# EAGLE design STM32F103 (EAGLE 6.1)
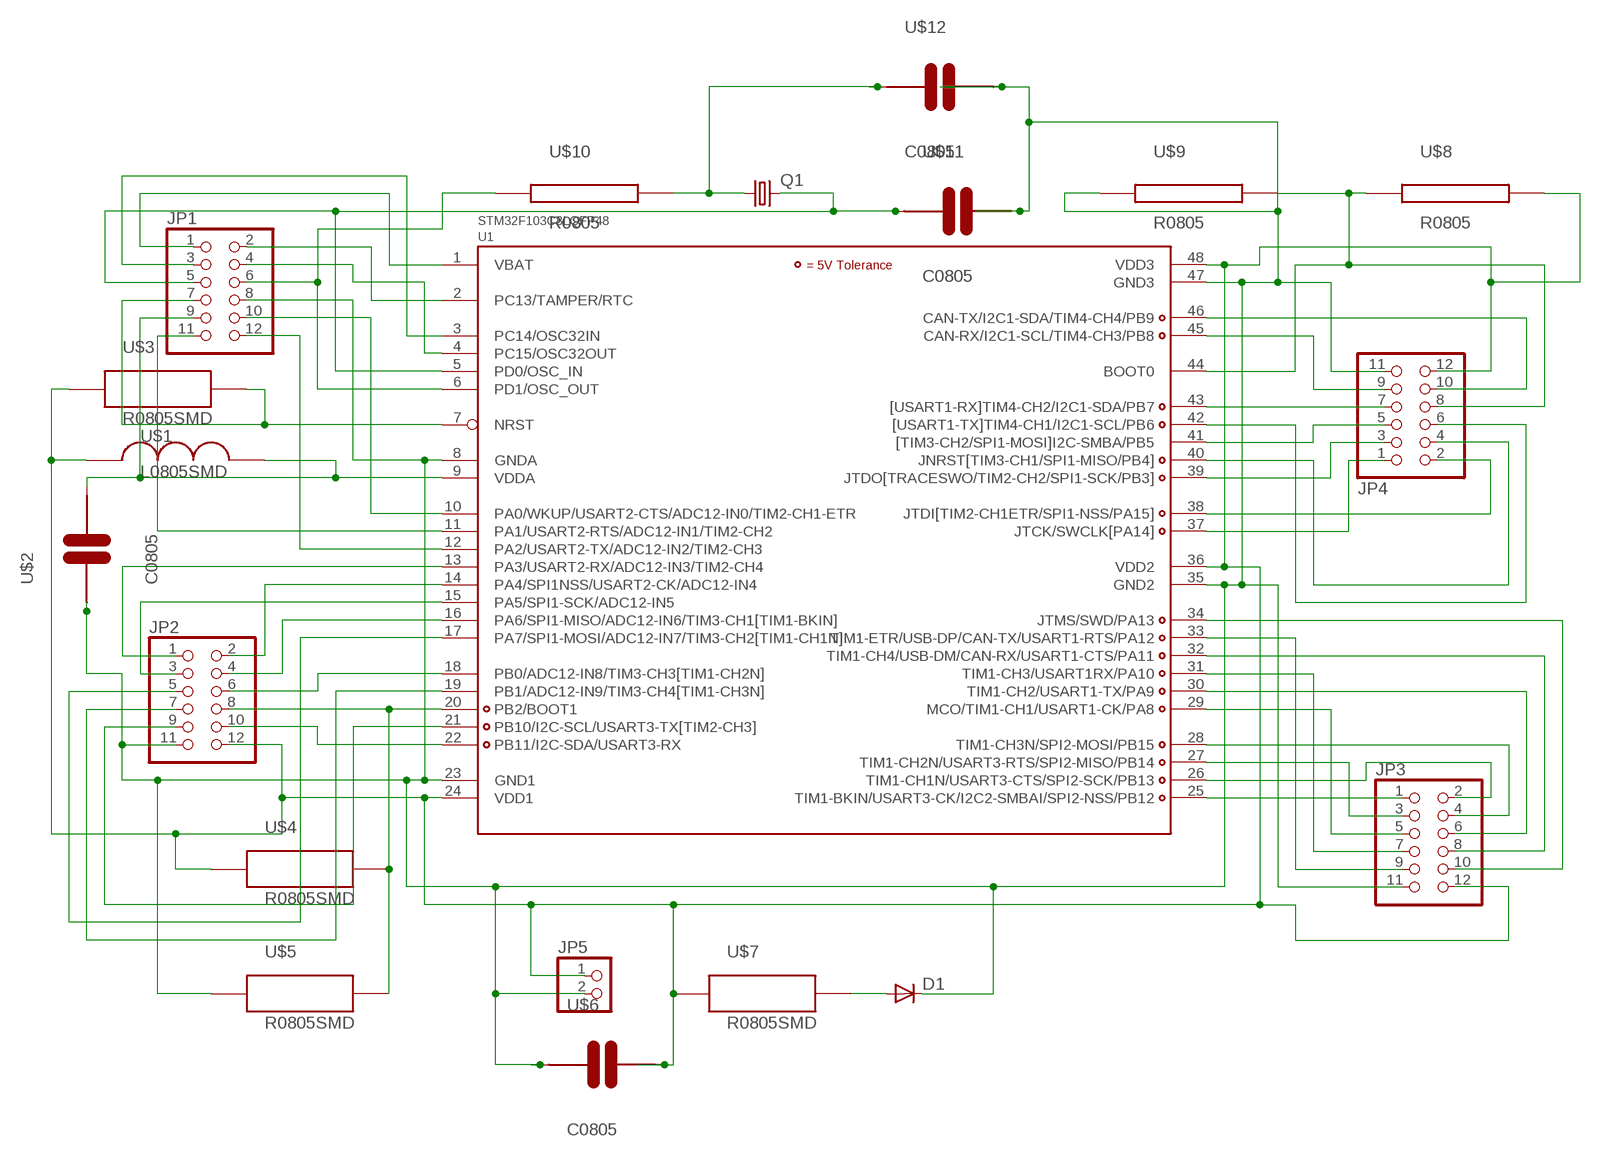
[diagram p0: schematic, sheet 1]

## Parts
D1  DIODE-DO214BA  [DO214BA]
JP1  PINHD-2X6  [2X06]
JP2  PINHD-2X6  [2X06]
JP3  PINHD-2X6  [2X06]
JP4  PINHD-2X6  [2X06]
JP5  PINHD-1X2  [1X02]
Q1  CRYSTALHC49U70  [HC49U70]
U1  STM32F103C8LQFP48  [LQFP48]
U$1  L0805SMD  [SMD0805]
U$2  C0805  [C0805]
U$3  R0805SMD  [SMD0805]
U$4  R0805SMD  [SMD0805]
U$5  R0805SMD  [SMD0805]
U$6  C0805  [C0805]
U$7  R0805SMD  [SMD0805]
U$8  R0805  [SMD0805]
U$9  R0805  [SMD0805]
U$10  R0805  [SMD0805]
U$11  C0805  [C0805]
U$12  C0805  [C0805]

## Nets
N$1: JP2.1 U1.13(PA3/USART2-RX/ADC12-IN3/TIM2-CH4)
N$2: JP1.2 U1.2(PC13/TAMPER/RTC)
N$3: JP1.3 U1.3(PC14/OSC32IN)
N$4: JP1.4 U1.4(PC15/OSC32OUT)
N$5: JP1.5 Q1.2 U1.5(PD0/OSC_IN) U$11.1
N$6: JP1.6 U1.6(PD1/OSC_OUT) U$10.1
N$7: JP1.7 U1.7(NRST) U$3.2
N$8: JP1.10 U1.10(PA0/WKUP/USART2-CTS/ADC12-IN0/TIM2-CH1-ETR)
N$9: JP1.11 U1.11(PA1/USART2-RTS/ADC12-IN1/TIM2-CH2)
N$10: JP1.12 U1.12(PA2/USART2-TX/ADC12-IN2/TIM2-CH3)
N$11: JP2.2 U1.14(PA4/SPI1NSS/USART2-CK/ADC12-IN4)
N$12: JP2.3 U1.15(PA5/SPI1-SCK/ADC12-IN5)
N$13: JP2.4 U1.16(PA6/SPI1-MISO/ADC12-IN6/TIM3-CH1[TIM1-BKIN])
N$14: JP2.5 U1.17(PA7/SPI1-MOSI/ADC12-IN7/TIM3-CH2[TIM1-CH1N])
N$15: JP2.6 U1.18(PB0/ADC12-IN8/TIM3-CH3[TIM1-CH2N])
N$16: JP2.7 U1.19(PB1/ADC12-IN9/TIM3-CH4[TIM1-CH3N])
N$17: JP2.8 U1.20(PB2/BOOT1) U$4.2 U$5.2
N$18: JP2.9 U1.21(PB10/I2C-SCL/USART3-TX[TIM2-CH3])
N$19: JP2.10 U1.22(PB11/I2C-SDA/USART3-RX)
N$20: JP3.1 U1.25(TIM1-BKIN/USART3-CK/I2C2-SMBAI/SPI2-NSS/PB12)
N$21: JP3.2 U1.26(TIM1-CH1N/USART3-CTS/SPI2-SCK/PB13)
N$22: JP3.3 U1.27(TIM1-CH2N/USART3-RTS/SPI2-MISO/PB14)
N$23: JP3.4 U1.28(TIM1-CH3N/SPI2-MOSI/PB15)
N$24: JP3.5 U1.29(MCO/TIM1-CH1/USART1-CK/PA8)
N$25: JP3.6 U1.30(TIM1-CH2/USART1-TX/PA9)
N$26: JP3.7 U1.31(TIM1-CH3/USART1RX/PA10)
N$27: JP3.8 U1.32(TIM1-CH4/USB-DM/CAN-RX/USART1-CTS/PA11)
N$28: JP3.9 U1.33(TIM1-ETR/USB-DP/CAN-TX/USART1-RTS/PA12)
N$29: JP3.10 U1.34(JTMS/SWD/PA13)
N$30: JP4.1 U1.37(JTCK/SWCLK[PA14])
N$31: JP4.2 U1.38(JTDI[TIM2-CH1ETR/SPI1-NSS/PA15])
N$32: JP4.3 U1.39(JTDO[TRACESWO/TIM2-CH2/SPI1-SCK/PB3])
N$33: JP4.4 U1.40(JNRST[TIM3-CH1/SPI1-MISO/PB4])
N$34: JP4.5 U1.41([TIM3-CH2/SPI1-MOSI]I2C-SMBA/PB5)
N$35: JP4.6 U1.42([USART1-TX]TIM4-CH1/I2C1-SCL/PB6)
N$36: JP4.7 U1.43([USART1-RX]TIM4-CH2/I2C1-SDA/PB7)
N$37: JP4.8 U1.44(BOOT0) U$8.1 U$9.2
N$38: JP4.9 U1.45(CAN-RX/I2C1-SCL/TIM4-CH3/PB8)
N$39: JP4.10 U1.46(CAN-TX/I2C1-SDA/TIM4-CH4/PB9)
N$50: Q1.1 U$10.2 U$12.1
N$54: D1.A U$7.2
N$68: JP2.12 JP3.12 JP4.12 JP5.1 U1.24(VDD1) U1.36(VDD2) U1.48(VDD3) U$1.1 U$3.1 U$4.1 U$6.2 U$7.1 U$8.2
N$80: D1.C JP1.8 JP2.11 JP3.11 JP4.11 JP5.2 U1.8(GNDA) U1.23(GND1) U1.35(GND2) U1.47(GND3) U$2.1 U$5.1 U$6.1 U$9.1 U$11.2 U$12.2
VBAT: JP1.1 U1.1(VBAT)
VDDA: JP1.9 U1.9(VDDA) U$1.2 U$2.2

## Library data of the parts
D1 = diode:DIODE-: DIODE
JP1-JP4 = pinhead:PINHD-2X6: PIN HEADER
JP5 = pinhead:PINHD-1X2: PIN HEADER
Q1 = crystal:CRYSTAL: CRYSTAL
U1 = STM32:STM32F103C8
U$1 = cansat1:L0805SMD: indukcnost v provedeni SMD0805
U$2 U$6 U$11 U$12 = cansat1:C0805: kondenzator v provedeni SMD0805
U$3-U$5 U$7 = cansat1:R0805SMD: REZISTOR v provedeni SMD0805
U$8-U$10 = cansat1:R0805: REZISTOR v provedeni SMD0805

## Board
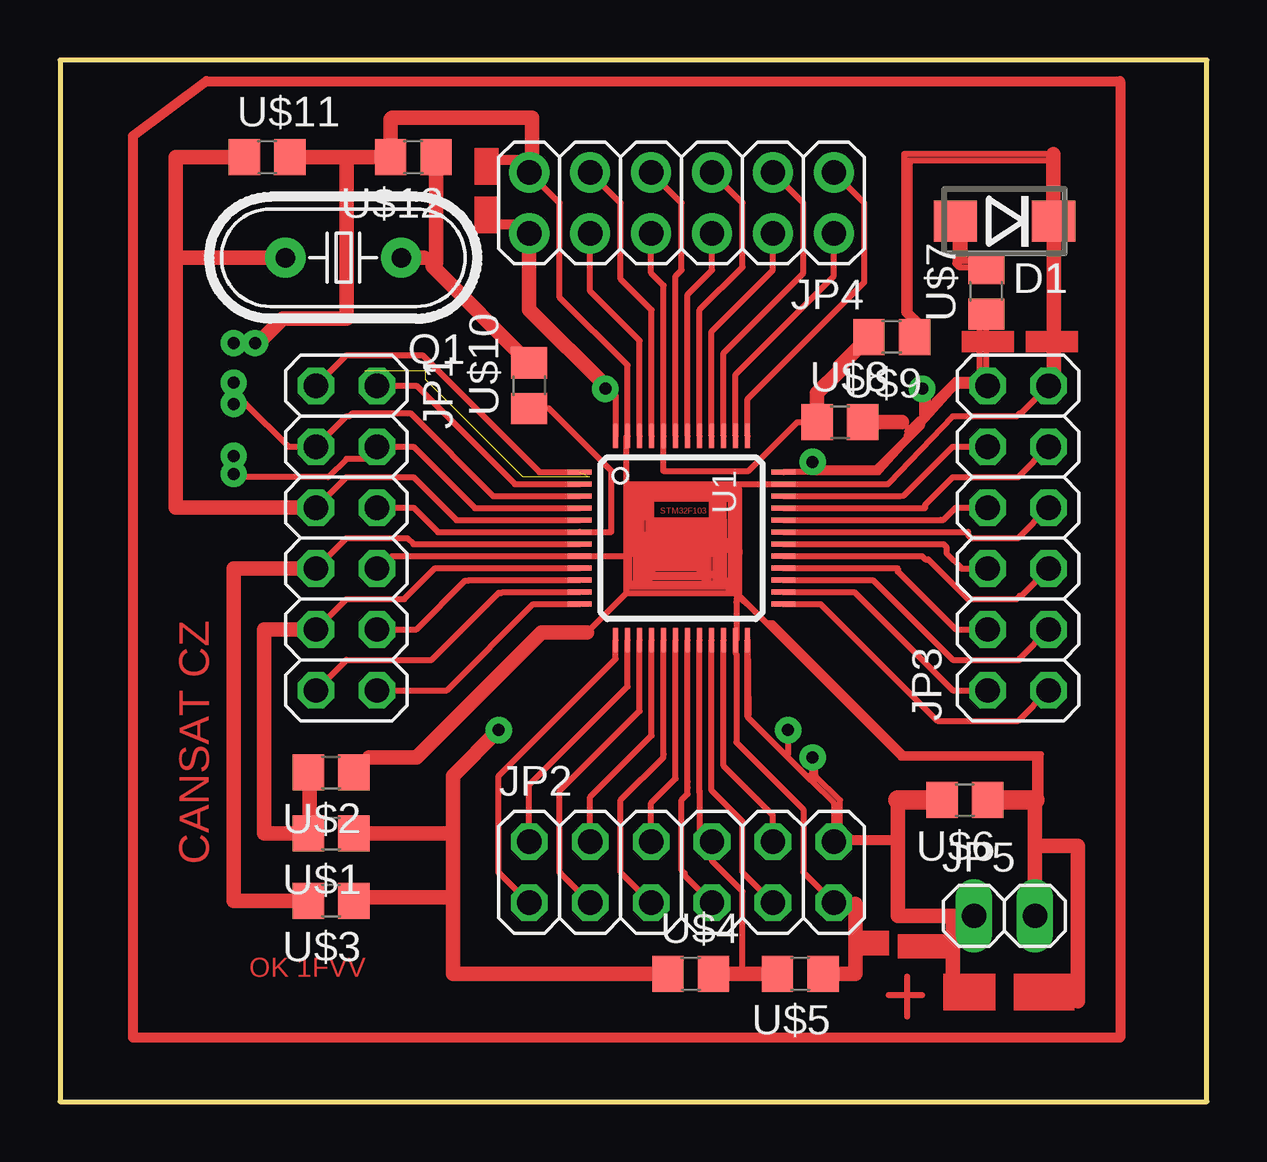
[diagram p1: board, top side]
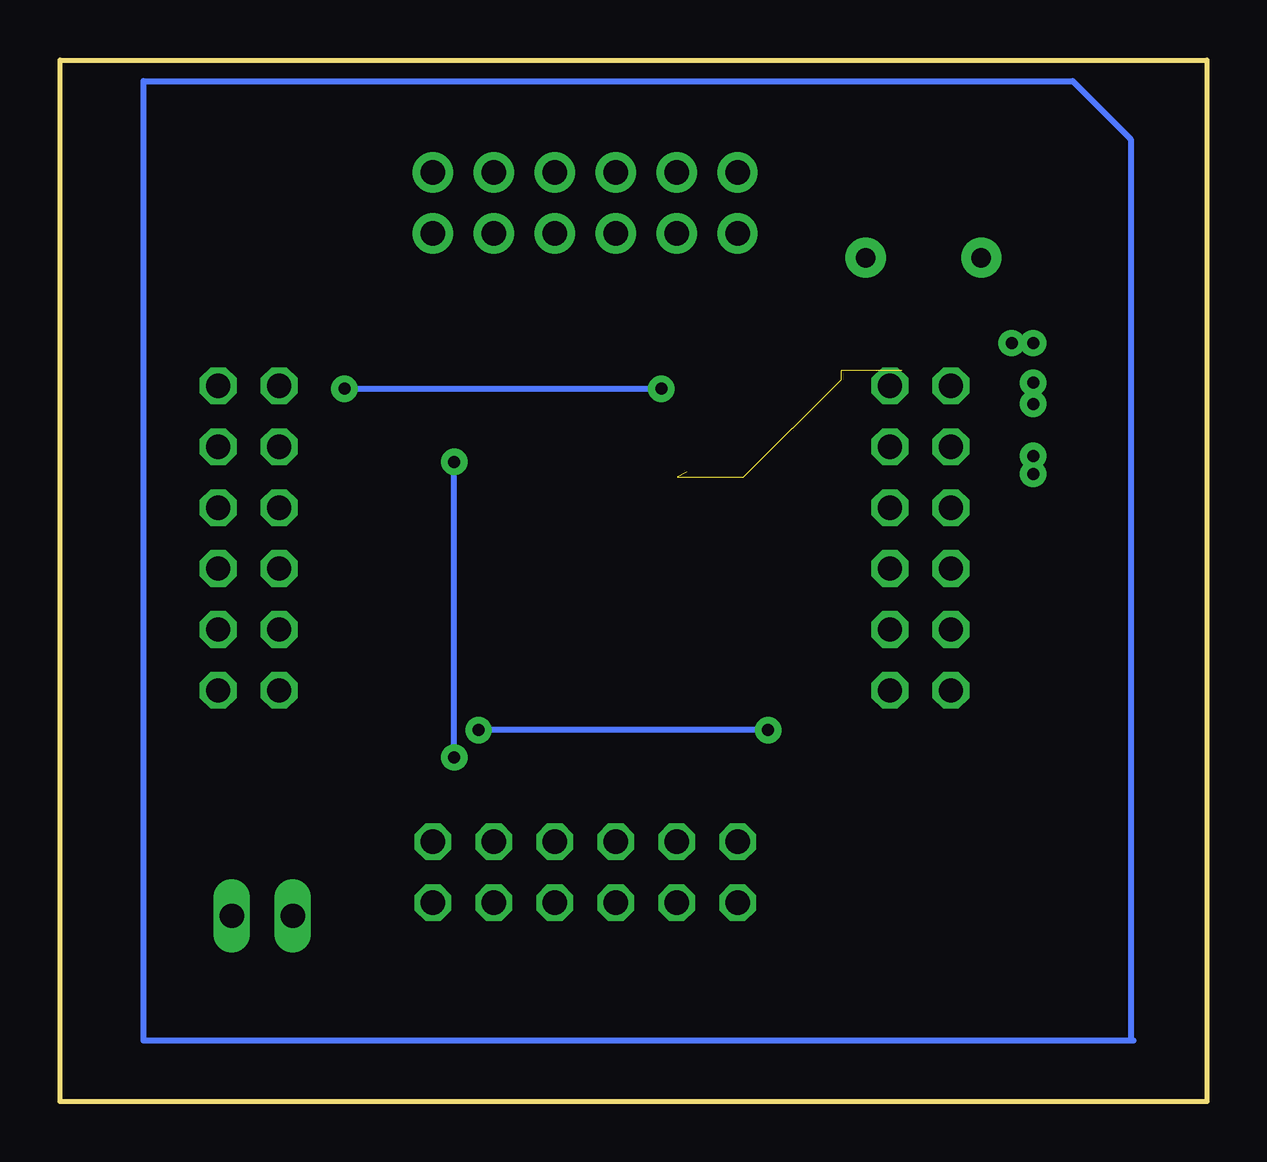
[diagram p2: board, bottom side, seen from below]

Size 47.8 x 43.42 mm. Coordinates in mm from the lower left corner, seen from the top.
Outline: 0,0 47.8,0 47.8,43.42 0,43.42 0,0
Copper layers (1*16): Top 0.035mm / dielectric 1.5mm / Bottom 0.035mm
Design rules: minimum track width 0.2mm, minimum drill 0.6mm, track to track 0.2mm, track to pad 0.2mm, pad to pad 0.2mm, via to via 0.2mm, smd to smd 8mil, copper to edge 40mil, drill to drill 2mm, minimum pad ring 0.2mm, minimum via ring 0.3mm, stop-mask expansion 4mil, vias tented up to drill 0mil, thermal gap 10mil

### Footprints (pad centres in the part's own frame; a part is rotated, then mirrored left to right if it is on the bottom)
DO214BA = smd 1.8 x 1.7: A 2.05,0; C -2.05,0
2X06 = drill 1.016 octagon: 1 -6.35,-1.27; 2 -6.35,1.27; 3 -3.81,-1.27; 4 -3.81,1.27; 5 -1.27,-1.27; 6 -1.27,1.27; 7 1.27,-1.27; 8 1.27,1.27; 9 3.81,-1.27; 10 3.81,1.27; 11 6.35,-1.27; 12 6.35,1.27
1X02 = drill 1.016 long: 1 -1.27,0; 2 1.27,0
HC49U70 = drill 0.813: 1 -2.413,0; 2 2.413,0
LQFP48 = smd 0.2 x 1: 1 -2.75,-4.25; 2 -2.25,-4.25; 3 -1.75,-4.25; 4 -1.25,-4.25; 5 -0.75,-4.25; 6 -0.25,-4.25; 7 0.25,-4.25; 8 0.75,-4.25; 9 1.25,-4.25; 10 1.75,-4.25; 11 2.25,-4.25; 12 2.75,-4.25; 25 2.75,4.25; 26 2.25,4.25; 27 1.75,4.25; 28 1.25,4.25; 29 0.75,4.25; 30 0.25,4.25; 31 -0.25,4.25; 32 -0.75,4.25; 33 -1.25,4.25; 34 -1.75,4.25; 35 -2.25,4.25; 36 -2.75,4.25 | smd 1 x 0.2: 13 4.25,-2.75; 14 4.25,-2.25; 15 4.25,-1.75; 16 4.25,-1.25; 17 4.25,-0.75; 18 4.25,-0.25; 19 4.25,0.25; 20 4.25,0.75; 21 4.25,1.25; 22 4.25,1.75; 23 4.25,2.25; 24 4.25,2.75; 37 -4.25,2.75; 38 -4.25,2.25; 39 -4.25,1.75; 40 -4.25,1.25; 41 -4.25,0.75; 42 -4.25,0.25; 43 -4.25,-0.25; 44 -4.25,-0.75; 45 -4.25,-1.25; 46 -4.25,-1.75; 47 -4.25,-2.25; 48 -4.25,-2.75
SMD0805 = smd 1.3 x 1.5: 1 -0.95,0; 2 0.95,0
C0805 = smd 1.3 x 1.5: 1 -0.95,0; 2 0.95,0

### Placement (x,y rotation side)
D1  39.37,36.7 180 top
JP1  11.94,23.49 270 top
JP2  25.91,9.56 0 top
JP3  39.94,23.49 90 top
JP4  25.91,37.46 180 top
JP5  39.37,7.75 0 top
Q1  11.81,35.18 180 top
U1  25.91,23.49 270 top
U$1  11.3,11.18 180 top
U$2  11.3,13.72 180 top
U$3  11.3,8.38 180 top
U$4  26.29,5.33 0 top
U$5  30.86,5.33 180 top
U$6  37.72,12.57 180 top
U$7  38.61,33.78 90 top
U$8  32.51,28.32 0 top
U$9  34.67,31.88 180 top
U$10  19.56,29.84 90 top
U$11  8.64,39.37 0 top
U$12  14.73,39.37 180 top

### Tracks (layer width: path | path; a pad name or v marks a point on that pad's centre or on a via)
N$1
  Top 0.254: JP2.1 18.33,9.53 18.29,9.53 18.29,13.59 23.16,18.46 U1.13
N$2
  Top 0.254: JP1.2 14.86,29.84 18.96,25.74 U1.2
N$3
  Top 0.254: JP1.3 11.94,28.57 12.06,28.57 12.19,28.7 14.61,28.7 18.06,25.24 U1.3
N$4
  Top 0.254: U1.4 17.29,24.74 14.73,27.3 JP1.4 12.7,26.8 11.94,26.8 11.18,26.03 7.62,26.03
N$5
  Top 0.254: JP1.5 11.94,26.03 14.73,26.03 16.52,24.24 U1.5
  Top 0.61: 4.83,35.18 Q1.2 | 4.83,35.18 4.83,24.77 JP1.5 | 4.83,35.18 4.83,39.37 U$11.1
N$6
  Top 0.254: JP1.6 14.73,24.77 15.75,23.74 U1.6 22.99,23.75 22.99,26.29 20.38,28.89 U$10.1
N$7
  Top 0.254: JP1.7 11.94,23.49 14.48,23.49 14.73,23.24 15.37,23.24 U1.7
  Top 0.61: JP1.7 7.24,22.23 7.24,8.38 U$3.2
N$8
  Top 0.254: JP1.10 14.86,19.69 16.89,21.72 17.02,21.72 17.05,21.74 U1.10
N$9
  Top 0.254: JP1.11 11.94,18.41 15.49,18.41 18.29,21.21 18.41,21.21 18.45,21.24 U1.11
N$10
  Top 0.254: JP1.12 16.13,17.14 19.73,20.74 U1.12
N$11
  Top 0.254: JP2.2 19.56,13.21 23.66,17.31 U1.14
N$12
  Top 0.254: JP2.3 20.87,9.53 20.83,9.53 20.83,12.95 24.16,16.28 U1.15
N$13
  Top 0.254: JP2.4 22.1,12.7 24.66,15.26 U1.16
N$14
  Top 0.254: JP2.5 23.37,9.56 23.37,12.57 25.15,14.35 25.15,14.48 25.16,14.49 U1.17
N$15
  Top 0.254: JP2.6 24.64,12.45 25.66,13.47 U1.18
N$16
  Top 0.254: U1.19 26.16,13.33 26.16,13.08 26.16,12.83 25.91,12.57 25.91,9.65 26.04,9.53 26.04,9.44 JP2.7
N$17
  Top 0.254: 26.67,11.47 JP2.8 | 26.67,11.47 26.67,12.83 26.66,12.94 U1.20 | 26.67,11.47 26.67,11.3 27.18,10.79 27.18,10.03 28.45,8.76 28.45,5.33
  Top 0.61: U$4.2 28.45,5.33 U$5.2
N$18
  Top 0.254: JP2.9 28.45,9.56 28.45,11.68 27.16,12.97 U1.21
N$19
  Top 0.254: JP2.10 29.72,11.94 27.66,14 U1.22
N$20
  Top 0.254: JP3.1 39.94,15.87 36.58,15.87 31.71,20.74 U1.25
N$21
  Top 0.254: JP3.2 37.21,17.14 33.11,21.24 U1.26
N$22
  Top 0.254: JP3.3 40.01,18.48 40.01,18.41 37.21,18.41 33.88,21.74 U1.27
N$23
  Top 0.254: JP3.4 37.34,19.69 34.92,22.1 34.92,22.23 34.91,22.24 U1.28
N$24
  Top 0.254: JP3.5 40.06,21.08 40.01,21.08 39.88,20.95 37.85,20.95 36.2,22.61 36.07,22.61 35.93,22.74 U1.29
N$25
  Top 0.254: JP3.6 37.59,22.23 36.96,22.86 36.96,23.11 36.83,23.24 U1.30
N$26
  Top 0.254: JP3.7 39.94,23.49 37.97,23.49 37.85,23.62 37.85,23.75 37.84,23.74 U1.31
N$27
  Top 0.254: JP3.8 37.34,24.77 36.83,24.26 36.7,24.26 36.69,24.24 U1.32
N$28
  Top 0.254: JP3.9 39.94,26.03 37.21,26.03 36.07,24.89 36.07,24.77 36.05,24.74 U1.33
N$29
  Top 0.254: JP3.10 37.21,27.3 35.18,25.27 35.02,25.24 U1.34
N$30
  Top 0.254: JP4.1 33.53,37.46 33.53,34.16 28.66,29.29 U1.37
N$31
  Top 0.254: JP4.2 32.26,34.42 28.16,30.32 U1.38
N$32
  Top 0.254: JP4.3 30.99,37.46 30.99,34.54 27.66,31.21 U1.39
N$33
  Top 0.254: JP4.4 29.72,34.67 27.16,32.11 U1.40
N$34
  Top 0.254: JP4.5 28.45,37.46 28.45,34.8 26.66,33.01 U1.41
N$35
  Top 0.254: JP4.6 27.18,34.67 26.16,33.65 U1.42
N$36
  Top 0.254: JP4.7 25.91,37.46 25.91,34.67 25.66,34.42 U1.43
N$37
  Top 0.254: JP4.8 24.64,34.54 25.16,34.02 U1.44 25.16,26.3 25.15,26.29 28.7,26.29 30.73,28.32 U$8.1 | 32.51,30.48 32.51,30.67
  Top 0.61: U$8.1 31.56,29.53 32.51,30.48 | 32.51,30.67 U$9.2
N$38
  Top 0.254: JP4.9 23.37,37.46 23.37,34.29 24.66,33 U1.45
N$39
  Top 0.254: JP4.10 22.1,33.78 24.16,31.72 U1.46
N$40  (via drill 0.7 pad 1.68)
  other vias: 19.56,36.2
N$41
  Top 0.254: 24.13,23.62 27.56,23.62 27.56,23.49 24.51,23.49 | 24.51,23.49 24.13,23.49 | 24.51,24.26 24.51,23.49 | 24.51,24.26 24.51,25.02 24.64,25.02 24.64,23.75 | 23.88,25.53 23.88,25.65 23.75,25.65 23.75,23.11 23.88,23.11 23.88,25.4 | 23.88,25.53 28.19,25.53 28.19,23.11 28.07,23.11 28.07,25.27 24,25.27 | 23.88,25.4 23.88,25.53 | 24,25.4 24.26,25.4 | 24,25.4 23.88,25.4 | 24,25.27 24,25.4 | 24,25.27 24,23.11 27.94,23.11 27.94,25.15 24.26,25.15 24.26,23.24 27.81,23.24 27.81,23.37 27.69,23.37 27.69,24.26 | 27.69,24.26 27.69,25.02 | 24.51,24.26 27.18,24.26 | 27.18,24.26 27.69,24.26 | 27.18,24.26 27.18,25.02 27.3,25.02 | 27.3,25.02 27.56,25.02 | 27.3,25.02 27.3,24.38 27.56,24.38 | 27.56,24.38 27.56,24.89 | 27.56,24.38 27.56,23.75 24.89,23.75 24.89,24.13 27.43,24.13 27.43,23.88 25.02,23.88 25.02,24 25.15,24
N$42
  Top 0.254: 24.51,23.37 27.43,23.37
N$43  (via drill 0.7 pad 1.68)
  other vias: 29.72,36.2
N$44  (via drill 0.7 pad 1.68)
  other vias: 24.64,36.2
N$45  (via drill 0.7 pad 1.68)
  other vias: 32.26,36.2
N$46  (via drill 0.7 pad 1.68)
  other vias: 27.18,36.2
N$47  (via drill 0.7 pad 1.68)
  other vias: 22.1,36.2
N$48  (via drill 0.7 pad 1.68)
  other vias: 9.4,35.18
N$49  (via drill 0.7 pad 1.68)
  other vias: 19.56,38.73
N$50
  Top 0.254: 15.17,35.18 15.52,34.83 15.68,34.99
  Top 0.61: Q1.1 15.17,35.18 | 15.52,34.83 U$10.2 | 15.68,34.99 U$12.1
N$51  (via drill 0.7 pad 1.68)
  other vias: 22.1,38.73
N$52  (via drill 0.7 pad 1.68)
  other vias: 24.64,38.73
N$53  (via drill 0.5 pad 0.81)
  other vias: 7.24,26.16
N$54
  Top 0.254: D1.A 37.32,34.94 37.46,34.8 38.54,34.8 U$7.2
N$55  (via drill 0.5 pad 0.81)
  other vias: 7.24,26.92
N$56  (via drill 0.5 pad 0.81)
  other vias: 7.24,29.08
N$57  (via drill 0.5 pad 0.81)
  other vias: 7.24,29.97
N$58  (via drill 0.5 pad 0.81)
  other vias: 7.24,31.62
N$59  (via drill 0.5 pad 0.81)
  other vias: 8.13,31.62
N$60
  Top 0.254: 7.11,29.59 7.75,29.08 9.53,27.3 10.54,27.3
N$61
  Top 0.61: 8.38,31.75 9.27,32.64 11.94,32.64 11.94,39.24
N$62
  Top 0.254: 34.54,4.44 35.94,4.44
N$63
  Top 0.254: 35.31,5.21 35.31,3.56
N$64
  Top 0.254: 32.51,11.05 32.51,12.57 31.5,13.59 31.24,13.59
N$65
  Top 0.254: 31.5,13.46 31.5,13.97
N$66
  Top 0.254: 31.88,26.42 34.04,26.42 | 34.04,26.42 34.16,26.42 | 34.04,26.42 35.31,27.69 35.31,27.81
N$67
  Top 0.254: 36.07,28.7 36.2,28.83 36.2,29.59
N$68  (via drill 0.5 pad 0.81)
  Top 0.254: 36.32,28.83 36.45,28.96 36.45,29.21 37.34,30.1 38.61,30.1 | U1.48 23.16,29.42 22.8,29.78 v22.73,29.72 | 35.12,27.37 34.16,26.29 34.12,26.24 31.37,26.24 | 35.12,27.37 35.56,27.85 | 35.56,27.85 37.34,29.84 JP3.12 38.61,29.9 38.61,30.1 | 31.37,26.24 U1.36 | 31.31,13.4 32.26,12.45 JP2.12 32.34,10.92 | 30.29,14.41 31.31,13.4 | 30.29,14.41 28.66,16.05 U1.24 28.7,16.13 | 35.94,28.45 35.94,28.19 35.12,27.37 | 35.94,28.45 v35.94,29.72 | v31.37,26.67 31.37,26.24 | v31.37,14.35 31.37,13.46 31.31,13.4 | 12.06,11.05 12.19,11.18 U$1.1 | v30.35,15.49 30.35,14.48 30.29,14.41 | U$3.1 12.38,8.51 | 38.61,30.1 U$7.1 | 35.56,27.85 35.09,28.32 | 35.31,27.94 35.81,28.45 35.94,28.45 | 38.61,30.1 38.35,30.35 38.35,32.26
  Top 0.406: 32.34,10.92 34.92,10.92
  Top 0.61: JP4.12 19.56,33.02 22.8,29.78 | 16.38,11.18 U$1.1 | 16.38,11.18 16.38,13.59 v18.29,15.49 | 12.38,8.51 16.38,8.51 | 16.38,8.51 16.38,11.18 | U$4.1 16.38,5.33 16.38,8.51 | JP5.1 34.92,7.75 34.92,10.92 34.92,12.57 | 35.09,28.32 U$8.2
  Top 0.813: 34.92,12.57 U$6.2
  Bottom 0.254: v35.94,29.72 v22.73,29.72 | v31.37,14.35 v31.37,26.67 | v18.29,15.49 v30.35,15.49
N$69
  Top 0.254: 41.27,30.1 41.27,35.81
N$70
  Top 0.254: 37.59,35.81 37.46,35.69 37.46,34.92
N$71
  Top 0.254: 37.34,35.05 37.72,35.05 | 37.72,35.05 38.1,35.05 | 37.72,35.05 37.72,35.94
N$72
  Top 0.254: 35.31,39.24 41.15,39.24 | 41.15,39.24 41.27,39.24 | 41.15,39.24 41.27,39.12 41.27,37.34
N$73
  Bottom 0.254: 3.05,2.54 3.17,2.54 | 3.17,2.54 44.32,2.54 44.32,42.54 5.59,42.54 3.17,40.13 3.17,2.54
N$74  (via drill 0.7 pad 1.68)
  other vias: 27.18,38.73
N$75  (via drill 0.7 pad 1.68)
  other vias: 29.72,38.73
N$76  (via drill 0.7 pad 1.68)
  other vias: 32.26,38.73
N$77  (via drill 0.7 pad 1.68)
  other vias: 14.22,35.18
N$78
  Top 0.406: 6.1,42.54 44.2,42.54 44.2,2.67 3.05,2.67 3.05,40.26 6.1,42.54
N$79
  Top 0.61: 37.21,7.62 37.21,4.32
N$80
  Top 0.254: 40.89,12.7 40.89,14.48 35.18,14.48 | 35.18,14.48 35.05,14.48 | 35.18,14.48 29.72,19.94 29.46,19.94 | JP1.8 13.33,22.23 13.84,22.73 21.65,22.73 U1.8 21.66,22.73 23.62,22.73 | 23.62,22.73 23.62,22.99 | 23.62,25.74 U1.35 34.51,25.74 34.54,25.78 37.21,28.57 39.88,28.57 40.01,28.7 40.06,28.7 JP3.11 41.42,30.06 | 23.62,25.74 23.62,27.74 U1.47 23.66,30.7 20.83,33.53 20.83,37.46 JP4.11 19.68,38.86 | 28.32,22.99 28.19,20.83 28.19,19.24 U1.23 28.16,18.7 28.19,18.67 28.19,14.99 30.99,12.19 30.99,9.56 JP2.11 32.3,8.26 33.15,8.26 | 28.07,22.99 23.62,22.99 | 23.62,22.99 23.62,25.74 | 23.62,21.21 23.62,22.73 | 23.62,21.21 28.07,21.21 | 28.07,21.21 28.07,22.99 | 28.07,22.99 28.32,22.99 | 28.32,22.99 28.32,25.53 27.94,25.53 27.94,21.46 23.75,21.46 23.75,22.86 27.69,22.86 27.69,21.72 27.81,21.72 27.81,21.59 27.56,21.59 27.56,22.73 27.3,22.73 27.3,21.59 27.05,21.59 | 26.92,21.59 24,21.59 | 24,21.59 23.88,21.59 | 24,21.59 24,22.73 26.29,22.73 | 26.29,22.73 27.05,22.73 27.05,21.59 | 27.05,21.59 26.92,21.59 | 26.92,21.59 26.92,22.48 24.13,22.48 24.13,21.72 24.38,21.72 24.38,22.35 26.8,22.35 26.8,21.84 24.64,21.84 24.64,22.23 24.51,22.23 24.51,21.97 | 24.51,21.97 24.51,21.72 | 24.51,21.97 26.67,21.97 26.67,22.23 24.77,22.23 | U$2.1 12.89,14.35 | 21.97,19.56 23.62,21.21 | 40.64,12.57 40.64,14.35 35.05,14.35 29.46,19.94 | U$9.1 35.62,32.45 35.31,32.77 | 35.31,32.77 35.18,32.89 35.18,39.5 41.4,39.5 | D1.C 41.4,36.72 | 13.84,41.02 13.78,40.96 | 28.07,21.21 28.32,21.21 28.32,22.99 | 28.7,20.7 29.46,19.94 | 26.29,22.73 28.7,20.7 | 35.31,32.77 35.43,32.89 | 35.43,32.89 35.43,39.12 | 35.43,32.89 35.81,32.51 | 28.7,20.7 28.32,21.08
  Top 0.406: 40.64,10.92 40.77,10.67 40.64,10.79
  Top 0.61: 42.42,4.19 42.42,10.67 40.77,10.67 | 12.89,14.35 14.86,14.35 20.07,19.56 21.97,19.56 | U$5.1 33.15,5.33 33.15,8.26 | 40.64,12.57 40.64,10.92 40.64,10.79 JP5.2 | 41.42,30.06 D1.C | 41.4,36.72 41.4,39.5 | U$11.2 U$12.2 13.78,40.96 | 13.84,41.02 19.68,41.02 19.68,38.86
  Top 0.813: 40.64,12.57 U$6.1
N$81
  Top 0.406: 19.43,39.24 17.65,39.24 17.65,39.37
N$82
  Top 0.406: 17.91,36.58 19.68,36.58
VBAT  (5 unrouted)
  Top 0.254: JP1.1 11.94,31.11 15.11,31.11 19.98,26.24 U1.1
VDDA
  Top 0.254: U1.9 15.64,22.24 14.35,20.95 11.94,20.95 JP1.9 10.79,19.94 10.67,19.94 10.41,19.69 | U$1.2 10.41,11.18 | 10.41,13.72 U$2.2
  Top 0.61: 10.41,19.69 8.51,19.69 8.51,11.18 U$1.2 | 10.41,11.18 10.41,13.72
(copper drawn outside any net)
  shapes: Top area x10

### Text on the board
Top: STM32F103 | CANSAT CZ | OK 1FVV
